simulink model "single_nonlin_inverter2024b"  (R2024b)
settings: Solver=VariableStepAuto  StartTime=0.0  StopTime=tsim  FixedStep=Tstep  RelTol=1e-3
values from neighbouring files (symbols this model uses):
  Cdc1 = 5    [simulink_parameters_one_bus.m]    (also in nine_bus_parameters.m)
  Cf1 = 50e-6    (= 5e-05)    [simulink_parameters_one_bus.m]    (also in nine_bus_parameters.m)
  Lc1 = 0.00615    [simulink_parameters_one_bus.m]    (also in nine_bus_parameters.m = 0.0123)
  Ldc1 = 1    [simulink_parameters_one_bus.m]    (also in nine_bus_parameters.m)
  Lf1 = 1.35e-3    (= 0.00135)    [simulink_parameters_one_bus.m]    (also in nine_bus_parameters.m)
  rc1 = 0.3    [simulink_parameters_one_bus.m]    (also in nine_bus_parameters.m = 0.03)
  rdc1 = 28.86    [simulink_parameters_one_bus.m]    (also in nine_bus_parameters.m)
  rf1 = 1    [simulink_parameters_one_bus.m]    (also in nine_bus_parameters.m = 0.1)
  Vdc1 = 1e3    (= 1000)    [simulink_parameters_one_bus.m]    (also in nine_bus_parameters.m)
  Vtri = Vdc1./3    [simulink_parameters_one_bus.m]    (also in nine_bus_parameters.m = Vdc./2)
  x0 = x01    [mlinearize_noninv.m]    (also in onebus_nonlinsub.m; DemoMTI_Boolean_Index_MTI.m = [0.5 0.0000]; DemoMTI_EKF.m = [1;-1;0.5]; DemoMTI_hybridSystemsTankExamples.m = 30)

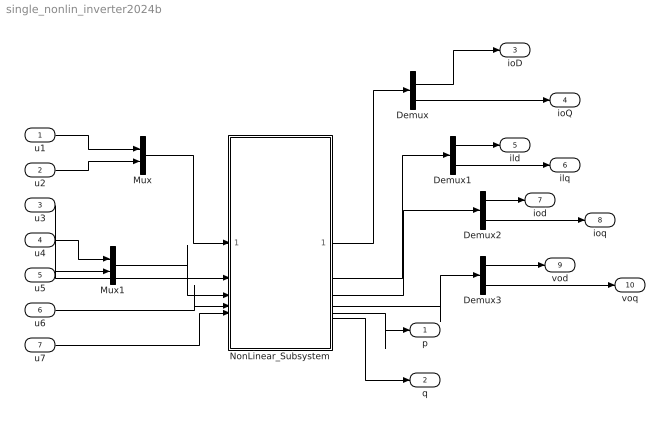
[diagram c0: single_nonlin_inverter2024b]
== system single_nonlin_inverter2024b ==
  u1 : Inport
  u2 : Inport  Port=2
  u3 : Inport  Port=3
  u4 : Inport  Port=4
  u5 : Inport  Port=5
  u6 : Inport  Port=6
  u7 : Inport  Port=7
  Demux{,1..3} (4 alike) : Demux  Outputs=2
  Mux : Mux  Inputs=2
  Mux1 : Mux  Inputs=2
  NonLinear_Subsystem : Subsystem
  p : Outport
  q : Outport  Port=2
  ioD : Outport  Port=3
  ioQ : Outport  Port=4
  ild : Outport  Port=5
  ilq : Outport  Port=6
  iod : Outport  Port=7
  ioq : Outport  Port=8
  vod : Outport  Port=9
  voq : Outport  Port=10
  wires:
  u1/1 -> Mux/1
  u2/1 -> Mux/2
  Mux/1 -> NonLinear_Subsystem/1(vbDQ)
  u4/1 -> Mux1/1
  u5/1 -> Mux1/2
  Mux1/1 -> NonLinear_Subsystem/3(vref)
  u3/1 -> NonLinear_Subsystem/2(P)
  u6/1 -> NonLinear_Subsystem/4(wi_in)
  u7/1 -> NonLinear_Subsystem/5(delta)
  NonLinear_Subsystem/5(p) -> p/1
  NonLinear_Subsystem/6(q) -> q/1
  NonLinear_Subsystem/1(ioDQ) -> Demux/1
  NonLinear_Subsystem/2(il) -> Demux1/1
  NonLinear_Subsystem/3(io) -> Demux2/1
  NonLinear_Subsystem/4(vo) -> Demux3/1
  Demux/1 -> ioD/1
  Demux/2 -> ioQ/1
  Demux1/1 -> ild/1
  Demux1/2 -> ilq/1
  Demux2/1 -> iod/1
  Demux2/2 -> ioq/1
  Demux3/1 -> vod/1
  Demux3/2 -> voq/1

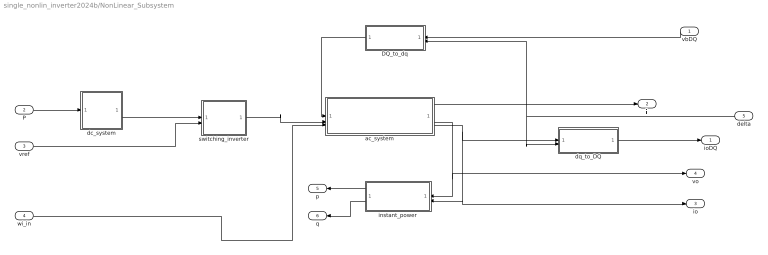
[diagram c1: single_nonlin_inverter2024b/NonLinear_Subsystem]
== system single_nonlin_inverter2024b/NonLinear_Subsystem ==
  vbDQ : Inport
  P : Inport  Port=2
  vref : Inport  Port=3
  wi_in : Inport  Port=4
  delta : Inport  Port=5
  DQ_to_dq : MATLAB Function  TreatAsAtomicUnit=on
  ac_system : Subsystem
  dc_system : Subsystem
  dq_to_DQ : MATLAB Function  TreatAsAtomicUnit=on
  instant_power : Subsystem
  switching_inverter : Subsystem
  ioDQ : Outport
  il : Outport  Port=2
  io : Outport  Port=3
  vo : Outport  Port=4
  p : Outport  Port=5
  q : Outport  Port=6
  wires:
  vref/1 -> switching_inverter/2(vref)
  P/1 -> dc_system/1(P)
  wi_in/1 -> ac_system/3(wi)
  dq_to_DQ/1(ioDQ) -> ioDQ/1
  ac_system/1(il) -> il/1
  ac_system/2(vo) -> vo/1, instant_power/1(vo)
  instant_power/1(p) -> p/1
  vbDQ/1 -> DQ_to_dq/1(vbDQ)
  instant_power/2(q) -> q/1
  switching_inverter/1(vl) -> ac_system/2(vl)
  DQ_to_dq/1(vbdq) -> ac_system/1(vb)
  delta/1 -> DQ_to_dq/2(delta), dq_to_DQ/2(delta)
  dc_system/1(vdc) -> switching_inverter/1(vdc)
  ac_system/3(io) -> dq_to_DQ/1(iodq), instant_power/2(io), io/1

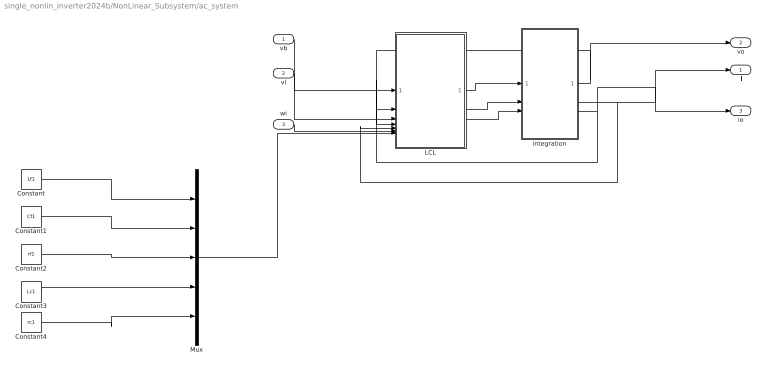
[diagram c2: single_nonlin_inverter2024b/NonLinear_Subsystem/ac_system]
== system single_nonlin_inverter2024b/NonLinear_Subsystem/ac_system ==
  vb : Inport
  vl : Inport  Port=2
  wi : Inport  Port=3
  Constant : Constant  Value=Lf1
  Constant1 : Constant  Value=Cf1
  Constant2 : Constant  Value=rf1
  Constant3 : Constant  Value=Lc1
  Constant4 : Constant  Value=rc1
  LCL : MATLAB Function  TreatAsAtomicUnit=on
  Mux : Mux  Inputs=5
  integration : Subsystem
  il : Outport  PortDimensions=[2 1]
  vo : Outport  Port=2  PortDimensions=[2 1]
  io : Outport  Port=3  PortDimensions=[2 1]
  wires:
  Mux/1 -> LCL/7(params)
  Constant4/1 -> Mux/5
  Constant3/1 -> Mux/4
  Constant2/1 -> Mux/3
  Constant1/1 -> Mux/2
  Constant/1 -> Mux/1
  integration/1(vo) -> LCL/2(vo), vo/1
  integration/3(io) -> LCL/4(io), io/1
  integration/2(il) -> il/1, LCL/5(il)
  LCL/3(dvo) -> integration/3(dvo)
  LCL/2(dio) -> integration/2(dio)
  LCL/1(dil) -> integration/1(dil)
  wi/1 -> LCL/6(wi)
  vb/1 -> LCL/1(vb)
  vl/1 -> LCL/3(vl)

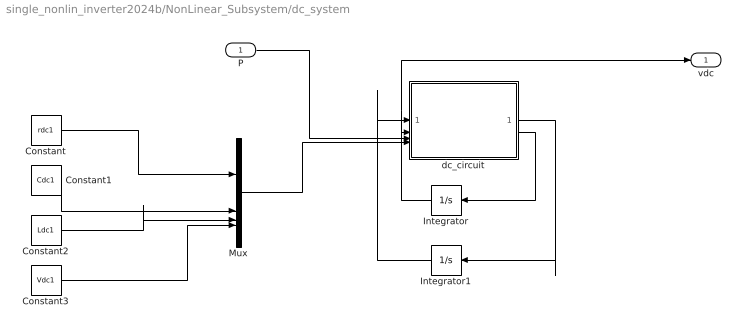
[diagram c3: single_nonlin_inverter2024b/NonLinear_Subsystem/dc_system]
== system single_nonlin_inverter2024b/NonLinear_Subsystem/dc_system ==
  P : Inport
  Constant : Constant  Value=rdc1
  Constant1 : Constant  Value=Cdc1
  Constant2 : Constant  Value=Ldc1
  Constant3 : Constant  Value=Vdc1
  Integrator : Integrator  InitialCondition=x0(2)
  Integrator1 : Integrator  InitialCondition=x0(1)
  Mux : Mux
  dc_circuit : MATLAB Function  TreatAsAtomicUnit=on
  vdc : Outport  PortDimensions=1
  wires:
  Constant3/1 -> Mux/4
  Constant2/1 -> Mux/3
  Constant1/1 -> Mux/2
  Mux/1 -> dc_circuit/4(params)
  Constant/1 -> Mux/1
  Integrator/1 -> dc_circuit/2(vdc), vdc/1
  dc_circuit/2(dvdc) -> Integrator/1
  P/1 -> dc_circuit/3(P)
  Integrator1/1 -> dc_circuit/1(idc)
  dc_circuit/1(didc) -> Integrator1/1

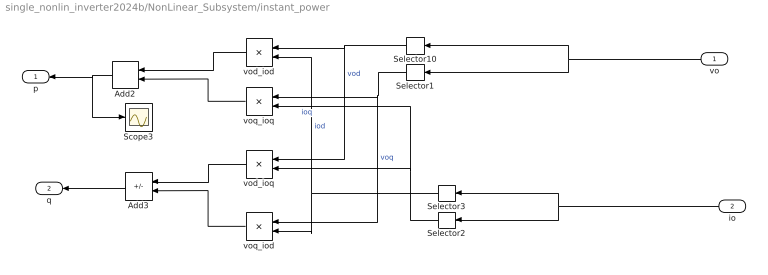
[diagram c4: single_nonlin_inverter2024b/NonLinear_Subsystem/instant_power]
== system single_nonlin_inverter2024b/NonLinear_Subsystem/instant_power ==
  vo : Inport
  io : Inport  Port=2
  Add2 : Sum
  Add3 : Sum  Inputs=+-
  Scope3 : Scope
  Selector1 : Selector  InputPortWidth=2  IndexOptions=Index vector (dialog)  Indices=2  OutputSizes=1
  Selector10 : Selector  InputPortWidth=2  IndexOptions=Index vector (dialog)  Indices=1  OutputSizes=1
  Selector2 : Selector  InputPortWidth=2  IndexOptions=Index vector (dialog)  Indices=2  OutputSizes=1
  Selector3 : Selector  InputPortWidth=2  IndexOptions=Index vector (dialog)  Indices=1  OutputSizes=1
  vod_iod : Product
  vod_ioq : Product
  voq_iod : Product
  voq_ioq : Product
  p : Outport
  q : Outport  Port=2
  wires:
  Add3/1 -> q/1
  Selector1/1 -> voq_ioq/1, voq_iod/1  "voq"
  vod_iod/1 -> Add2/1
  voq_ioq/1 -> Add2/2
  io/1 -> Selector3/1, Selector2/1
  voq_iod/1 -> Add3/2
  Add2/1 -> Scope3/1, p/1
  vod_ioq/1 -> Add3/1
  Selector10/1 -> vod_iod/1, vod_ioq/1  "vod"
  Selector3/1 -> vod_iod/2, voq_iod/2  "iod"
  vo/1 -> Selector1/1, Selector10/1
  Selector2/1 -> voq_ioq/2, vod_ioq/2  "ioq"

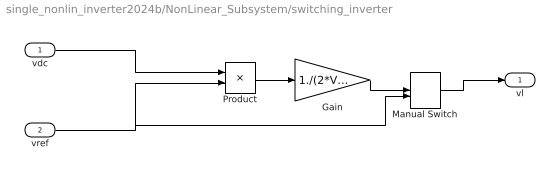
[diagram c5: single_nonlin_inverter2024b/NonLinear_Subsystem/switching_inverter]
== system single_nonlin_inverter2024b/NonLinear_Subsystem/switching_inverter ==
  vdc : Inport
  vref : Inport  Port=2
  Gain : Gain  Gain=1./(2*Vtri(1))
  Manual Switch : ManualSwitch
  Product : Product
  vl : Outport  PortDimensions=[2 1]
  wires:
  Manual Switch/1 -> vl/1
  Gain/1 -> Manual Switch/1
  vref/1 -> Product/2, Manual Switch/2
  vdc/1 -> Product/1
  Product/1 -> Gain/1

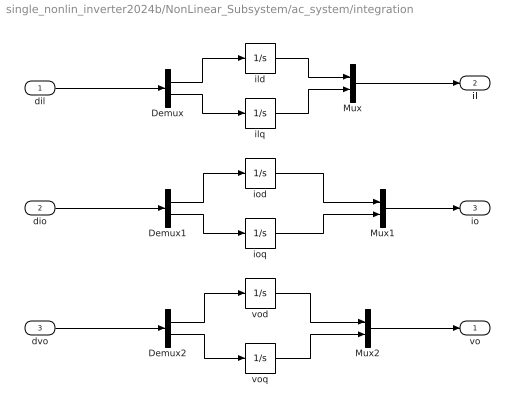
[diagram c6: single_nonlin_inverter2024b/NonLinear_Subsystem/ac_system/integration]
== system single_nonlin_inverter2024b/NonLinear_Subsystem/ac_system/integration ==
  dil : Inport
  dio : Inport  Port=2
  dvo : Inport  Port=3
  Demux : Demux  Outputs=2
  Demux1 : Demux  Outputs=2
  Demux2 : Demux  Outputs=2
  Mux : Mux  Inputs=2
  Mux1 : Mux  Inputs=2
  Mux2 : Mux  Inputs=2
  ild : Integrator  InitialCondition=x0(10)
  ilq : Integrator  InitialCondition=x0(11)
  iod : Integrator  InitialCondition=x0(14)
  ioq : Integrator  InitialCondition=x0(15)
  vod : Integrator  InitialCondition=x0(12)
  voq : Integrator  InitialCondition=x0(13)
  vo : Outport
  il : Outport  Port=2
  io : Outport  Port=3
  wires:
  dvo/1 -> Demux2/1
  dil/1 -> Demux/1
  Demux/2 -> ilq/1
  Demux/1 -> ild/1
  Mux2/1 -> vo/1
  Mux/1 -> il/1
  Demux1/2 -> ioq/1
  Demux2/2 -> voq/1
  Demux2/1 -> vod/1
  Mux1/1 -> io/1
  iod/1 -> Mux1/1
  dio/1 -> Demux1/1
  ioq/1 -> Mux1/2
  voq/1 -> Mux2/2
  ild/1 -> Mux/1
  vod/1 -> Mux2/1
  ilq/1 -> Mux/2
  Demux1/1 -> iod/1

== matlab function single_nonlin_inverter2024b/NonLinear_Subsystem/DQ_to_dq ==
function vbdq  = DQ_to_dq(vbDQ,delta)

vbdq = [cos(delta) sin(delta);-sin(delta) cos(delta)]*vbDQ;

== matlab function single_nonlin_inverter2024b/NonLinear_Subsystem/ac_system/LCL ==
function [dil,dio,dvo] = ac_circuit(vb,vo,vl,io,il,wi,params)
% 
Lf = params(1);   
Cf = params(2);   
rf = params(3); 
Lc = params(4); 
rc = params(5);

dil = -(rf/Lf).*il + wi.*[0 1;-1 0]*il + (1/Lf).*(vl-vo);
dio = -(rc/Lc).*io + wi.*[0 1;-1 0]*io + (1/Lc).*(vo-vb);
dvo = (1/Cf).*(il-io) + wi.*[0 1;-1 0]*vo;

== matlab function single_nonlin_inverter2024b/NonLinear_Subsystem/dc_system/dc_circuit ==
function[didc, dvdc] = dc_circuit(idc,vdc,P,params)

% rdc = 28.86;
% Cdc = 5;
% Ldc = 1;
% Vdc = 1000;
rdc = params(1);
Cdc = params(2);
Ldc = params(3);
Vdc = params(4);

dx = [-rdc/Ldc -1/Ldc;1/Cdc 0]*[idc;vdc] + [0;-1/(Cdc*vdc)]*P + [Vdc/Ldc;0];

didc = dx(1);
dvdc = dx(2);

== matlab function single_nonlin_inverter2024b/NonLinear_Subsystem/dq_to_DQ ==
function ioDQ  = dq_to_DQ(iodq,delta)

ioDQ = [cos(delta) -sin(delta);sin(delta) cos(delta)]*iodq;
